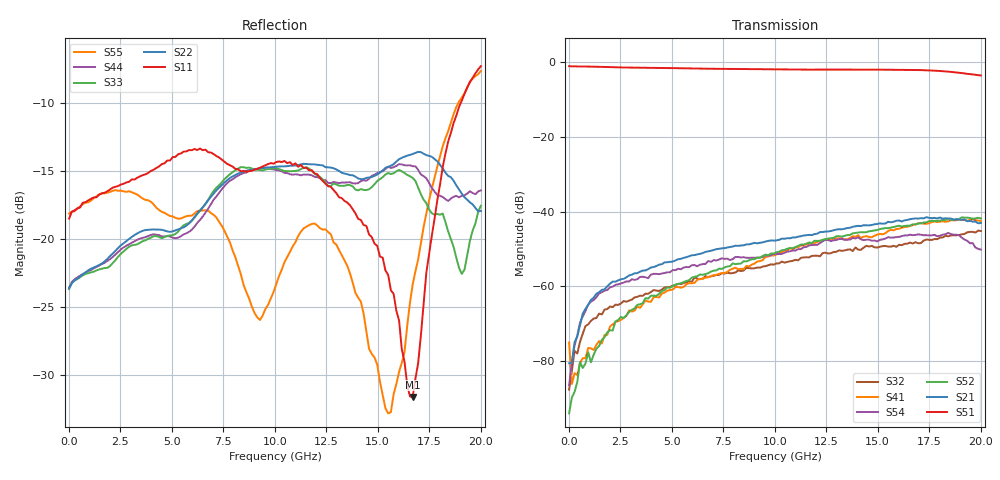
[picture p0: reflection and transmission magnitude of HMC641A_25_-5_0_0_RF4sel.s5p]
! Device:  HMC641A
! Description: GaAs MMIC SP4T NON-REFLECTIVE
! Frequency:  0.01 -  18 GHz
! Ports:
! RFC = Port 1
! RF1 = Port 2
! RF2 = Port 3
! RF3 = Port 4
! RF4 = Port 5
! State: RF4 selected
! Vss:  -5 Volts
! Control A  0 Volts
! Control B:  0 Volts
! Temperature = +85 C
! Data: Data was collected using a calibrated network analyzer.
!  The reference plane is the edge of the device.
! Note: Analog Devices supplies this data as a sample of measured data for this product.
!  Your particular data for this product may vary.
!  Analog Devices reserves the right to change this data at anytime
# Hz S DB R 50.0
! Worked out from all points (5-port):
!   152 points, 10 MHz to 20.01 GHz, reference 50 ohm
!   strongest paths, dB at 10 MHz, 5.043 GHz, 10.08 GHz, 15.11 GHz, 20.01 GHz:
!     S51: -1.1, -1.7, -2.0, -2.1, -3.6
!     S21: -80.6, -53.4, -47.7, -43.2, -43.1
!     S52: -94.0, -59.9, -50.9, -44.7, -41.9
!     S54: -86.4, -55.7, -51.3, -47.6, -50.2
!     S41: -75.0, -60.9, -51.5, -46.0, -42.5
!     S32: -87.7, -59.8, -53.9, -49.4, -45.2
!   lowest |S11| = -31.6 dB at 16.7 GHz (marker M1), VSWR 1.05, Z = 51.7 + j2.08 ohm
!   |S11| at or under -10 dB: start of sweep to 19.02 GHz
